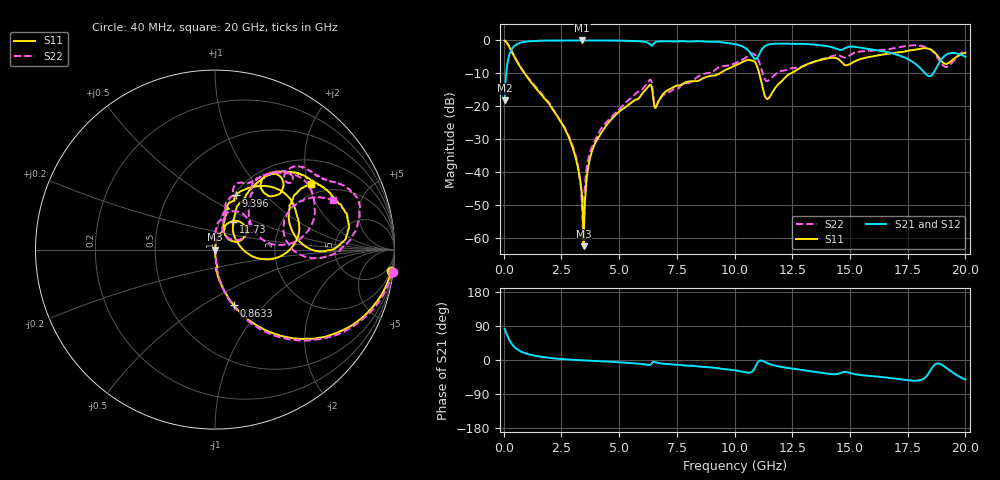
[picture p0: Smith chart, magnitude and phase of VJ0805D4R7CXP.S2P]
! VJ0805D4R7CXP
! DATE 10/29/2021  11:51
! CAPACITORS MOUNTED IN SERIES ON 25 MIL THICK MICROSTRIP SUBSTRATE
# GHz  S  MA  R  50.00
!  FREQ  S11M  S11A  S21M  S21A  S12M  S12A  S22M  S22A
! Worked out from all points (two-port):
!   1601 points, 40 MHz to 20 GHz, reference 50 ohm
!   highest |S21| = -0.02 dB at 3.396 GHz (marker M1); lowest = -18.3 dB at 40 MHz (marker M2)
!   |S21| within 3 dB of the highest: 321.9 MHz to 10.59 GHz (10.27 GHz wide, 188 % of centre); 11.16 GHz to 16.18 GHz (5.025 GHz wide, 36.8 % of centre)
!   lowest |S11| = -62.5 dB at 3.458 GHz (marker M3), VSWR 1.00, Z = 50.1 + j0.00978 ohm
!   |S11| at or under -10 dB: 896.6 MHz to 9.363 GHz (8.466 GHz wide, 165 % of centre); 11.07 GHz to 12.44 GHz (1.374 GHz wide, 11.7 % of centre)
!   |S22| runs from -57.4 to 0.0 dB; largest |S21 - S12| = 0.006
!   S11 on the Smith chart (normalised r, x): 40 MHz: 1, -16; 863.4 MHz: 1.00, -0.69; 9.396 GHz: 1.02, +0.69; 11.73 GHz: 1.16, +0.37; 20 GHz: 1.67, +2.10
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0.04  0.9907 -7.1  0.1223 82.6  0.1224 82.5  0.9976 -7.3
0.301975  0.7272 -43.1  0.6828 46.9  0.6831 46.8  0.7354 -43.4
0.86335  0.3287 -71.2  0.9449 19.3  0.9452 19.2  0.3389 -71.4
2.796975  0.03546 -86.9  0.9956 1.3  0.997 1.2  0.0372 -82.9
3.1837  0.01316 -79.8  0.9969 -0.1  0.9971 -0.2  0.01424 -81.3
3.370825  0.005259 -66.0  0.9975 -0.7  0.9977 -0.8  0.004276 -94.0
3.395775  0.004132 -61.8  0.9977 -0.8  0.9978 -0.9  0.00284 -107.0
3.45815  0.0007471 7.5  0.9971 -1.0  0.9975 -1.1  0.002399 140.9
3.7825  0.01858 84.2  0.9968 -2.0  0.9971 -2.1  0.02188 88.5
4.3813  0.04703 80.6  0.9948 -3.9  0.9959 -4.0  0.05402 86.4
6.30245  0.2063 49.6  0.8945 -13.2  0.8952 -13.3  0.2467 59.0
6.70165  0.1176 66.1  0.9647 -7.9  0.9654 -8.0  0.1172 68.8
9.39625  0.3226 69.2  0.9413 -22.9  0.9416 -23.0  0.4029 67.8
10.02  0.4133 57.9  0.8766 -27.3  0.8773 -27.5  0.4472 60.3
10.88077  0.4698 9.4  0.5224 -20.9  0.5225 -20.9  0.6047 23.4
11.3673  0.1325 15.7  0.8383 -6.8  0.8381 -7.0  0.2423 23.5
11.72907  0.1826 56.3  0.8902 -14.6  0.8905 -14.8  0.2965 50.6
13.35083  0.4627 56.6  0.8696 -30.2  0.8694 -30.4  0.4585 59.3
16.68165  0.6296 42.3  0.6535 -47.1  0.6541 -47.3  0.7356 31.5
18.02895  0.746 18.9  0.3856 -53.6  0.3849 -53.9  0.8295 14.1
18.76497  0.5982 -0.9  0.3983 -9.4  0.3987 -9.5  0.5687 -4.7
20  0.6493 34.1  0.5646 -51.6  0.5643 -52.0  0.7148 22.9
